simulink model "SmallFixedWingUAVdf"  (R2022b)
settings: Solver=ode4  StartTime=0  StopTime=stoptime  FixedStep=0.001  RelTol=1e-3  EnableMultiTasking=on
PreLoadFcn:
  | asbswarm_vehicledata; % load in workspace variables
PostLoadFcn:
  | open_system([gcs,'/MATLAB Animation Display/MATLAB',10,'Animation']);
InitFcn:
  | InitDatactrl
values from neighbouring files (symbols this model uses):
  uav = struct    [InitDatactrl.m]    (also in InitDatactrldf.m)
undefined symbols (not defined in the file or in its folder): Busy, Wait
libraries: aerolibptmass x1, aerolibanimutils x1

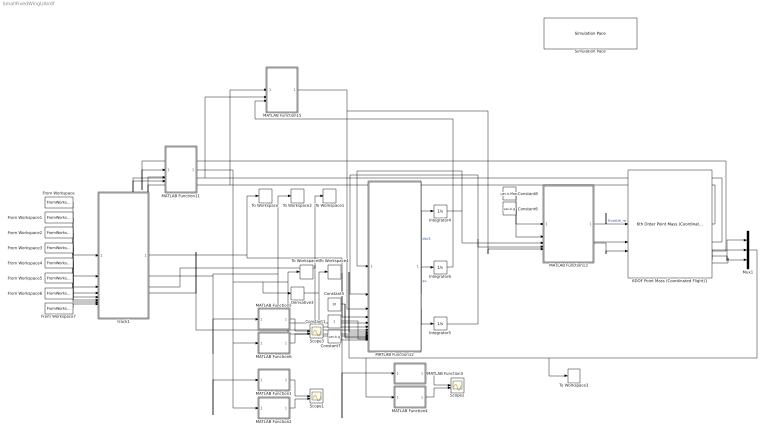
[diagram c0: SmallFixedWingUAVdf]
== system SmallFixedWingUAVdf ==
  6DOF Point Mass (Coordinated Flight)1 : aerolibptmass/6th Order Point Mass (Coordinated Flight)  units=Metric (MKS)  gamma0=uav.ic.Gam  chi0=uav.ic.Chi  V0=uav.ic.V  x0=uav.ic.East  y0=uav.ic.North  h0=uav.ic.Up  mass0=uav.ic.Mass
  Constant1 : Constant
  Constant5 : Constant  Value=10
  Constant6 : Constant  Value=uav.ic.g
  Constant7 : Constant  Value=uav.ic.g
  Constant8 : Constant  Value=uav.ic.Mass
  Derivative3 : Derivative
  From Workspace : FromWorkspace  VariableName=xts  SampleTime=-1
  From Workspace1 : FromWorkspace  VariableName=yts  SampleTime=-1
  From Workspace2 : FromWorkspace  VariableName=dxts  SampleTime=-1
  From Workspace3 : FromWorkspace  VariableName=dyts  SampleTime=-1
  From Workspace4 : FromWorkspace  VariableName=ddxts  SampleTime=-1
  From Workspace5 : FromWorkspace  VariableName=ddyts  SampleTime=-1
  From Workspace6 : FromWorkspace  VariableName=dddxts  SampleTime=-1
  From Workspace7 : FromWorkspace  VariableName=dddyts  SampleTime=-1
  Integrator4 : Integrator
  Integrator5 : Integrator
  Integrator6 : Integrator
  MATLAB Function1 : MATLAB Function  TreatAsAtomicUnit=on
  MATLAB Function11 : MATLAB Function  TreatAsAtomicUnit=on
  MATLAB Function12 : MATLAB Function  TreatAsAtomicUnit=on
  MATLAB Function13 : MATLAB Function  TreatAsAtomicUnit=on
  MATLAB Function15 : MATLAB Function  TreatAsAtomicUnit=on
  MATLAB Function2 : MATLAB Function  TreatAsAtomicUnit=on
  MATLAB Function3 : MATLAB Function  TreatAsAtomicUnit=on
  MATLAB Function4 : MATLAB Function  TreatAsAtomicUnit=on
  MATLAB Function5 : MATLAB Function  TreatAsAtomicUnit=on
  MATLAB Function6 : MATLAB Function  TreatAsAtomicUnit=on
  Mux1 : Mux  Inputs=3
  Scope1 : Scope  NumInputPorts=2
  Scope2 : Scope  NumInputPorts=2
  Scope3 : Scope  NumInputPorts=2
  Simulation Pace : aerolibanimutils/Simulation Pace  SimulationPace=1  SleepMode=Busy-Wait  OutputPaceError=off  SampleTime=-1
  To Workspace : ToWorkspace  VariableName=Xd  SampleTime=0.1
  To Workspace1 : ToWorkspace  VariableName=Ad  SampleTime=0.1
  To Workspace2 : ToWorkspace  VariableName=Vd  SampleTime=0.1
  To Workspace3 : ToWorkspace  VariableName=X  SampleTime=0.1
  To Workspace4 : ToWorkspace  VariableName=A  SampleTime=0.1
  To Workspace5 : ToWorkspace  VariableName=V  SampleTime=0.1
  track1 : MATLAB Function  TreatAsAtomicUnit=on
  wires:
  Constant5/1 -> MATLAB Function12/11(k1), MATLAB Function12/12(k2)
  Constant6/1 -> MATLAB Function13/2(g)
  Integrator5/1 -> MATLAB Function13/4(av3), MATLAB Function12/2(av3)
  MATLAB Function12/1(dav1) -> Integrator4/1  "dav1"
  Integrator4/1 -> MATLAB Function12/1(av1), MATLAB Function13/3(av1)
  Derivative3/1 -> To Workspace4/1, MATLAB Function12/10(ddx)
  MATLAB Function12/3(dav3) -> Integrator5/1
  Constant7/1 -> MATLAB Function12/14(g)
  MATLAB Function13/2(Fy) -> 6DOF Point Mass (Coordinated Flight)1/2
  MATLAB Function13/1(Fx) -> 6DOF Point Mass (Coordinated Flight)1/1  "throttle_re"
  MATLAB Function13/3(Fz) -> 6DOF Point Mass (Coordinated Flight)1/3
  Constant8/1 -> MATLAB Function13/1(m)
  6DOF Point Mass (Coordinated Flight)1/3 -> MATLAB Function11/1(Velocity)
  6DOF Point Mass (Coordinated Flight)1/1 -> MATLAB Function15/1(gamma), MATLAB Function11/2(gamma)
  6DOF Point Mass (Coordinated Flight)1/2 -> MATLAB Function15/2(chi), MATLAB Function11/3(chi)
  MATLAB Function11/1(dx) -> To Workspace5/1, MATLAB Function12/9(dx), Derivative3/1, MATLAB Function6/1(u), MATLAB Function2/1(u)
  MATLAB Function12/2(w1) -> Integrator6/1  "av"
  Integrator6/1 -> MATLAB Function15/3(mu)
  MATLAB Function15/1(R) -> MATLAB Function13/5(R), MATLAB Function12/3(R)
  MATLAB Function5/1(y) -> Scope3/1
  MATLAB Function6/1(y) -> Scope3/2
  MATLAB Function1/1(y) -> Scope1/1
  MATLAB Function2/1(y) -> Scope1/2
  6DOF Point Mass (Coordinated Flight)1/5 -> Mux1/2
  6DOF Point Mass (Coordinated Flight)1/6 -> Mux1/3
  6DOF Point Mass (Coordinated Flight)1/4 -> Mux1/1
  Mux1/1 -> To Workspace3/1, MATLAB Function12/8(x), MATLAB Function4/1(u)
  MATLAB Function4/1(y) -> Scope2/2
  MATLAB Function3/1(y) -> Scope2/1
  From Workspace/1 -> track1/1(x)
  From Workspace1/1 -> track1/2(y)
  From Workspace2/1 -> track1/3(dx)
  From Workspace3/1 -> track1/4(dy)
  From Workspace4/1 -> track1/5(ddx)
  From Workspace5/1 -> track1/6(ddy)
  From Workspace6/1 -> track1/7(dddx)
  From Workspace7/1 -> track1/8(dddy)
  track1/1(Xd) -> To Workspace/1, MATLAB Function12/4(xd), MATLAB Function3/1(u)
  track1/2(Vd) -> To Workspace2/1, MATLAB Function12/5(dxd), MATLAB Function1/1(u), MATLAB Function5/1(u)
  track1/3(Ad) -> To Workspace1/1, MATLAB Function12/6(ddxd)
  track1/4(Jd) -> MATLAB Function12/7(dddxd)
  Constant1/1 -> MATLAB Function12/13(k3)

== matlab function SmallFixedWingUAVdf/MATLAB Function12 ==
function [dav1,w1,dav3] = DF(av1,av3,R,xd,dxd,ddxd,dddxd,x,dx,ddx,k1,k2,k3,g)
    dav1=zeros(1,1);
    w1=zeros(1,1);
    dav3=zeros(1,1);
    
    V = norm(dx,2);
    gv = R'*[0;0;-g];
    w2=-(av3+gv(3))/V;
    w3=gv(2)/V;

    u = dddxd + k1*(ddxd-ddx) + k2*(dxd-dx)+ k3*(xd-x);

    a = [-w2*av3;w3*av1/av3;w2*av1];
    B = [1,0,0;0,-1/av3,0;0,0,1];
    out = a + B*R'*u;

    dav1=out(1); w1=out(2); dav3=out(3);

    if isnan(dav1)
        dav1=0;
    end
    if isnan(w1)
        w1=0;
    end
    if isnan(dav3)
        dav3=0;
    end

end

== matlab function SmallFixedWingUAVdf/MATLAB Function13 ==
function [Fx,Fy,Fz] = fcn(m,g,av1,av3,R)
N=3;
Fxyz=zeros(N,1);

av = [av1;0;av3];
a = [0;0;-g]+R*av;
Fxyz = R'*(m*a);
Fx=Fxyz(1);
Fy=Fxyz(2);
Fz=Fxyz(3);

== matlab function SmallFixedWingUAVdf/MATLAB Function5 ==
function y = fcn(u)

y = u(1);

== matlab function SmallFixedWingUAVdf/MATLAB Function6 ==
function y = fcn(u)

y = u(1);

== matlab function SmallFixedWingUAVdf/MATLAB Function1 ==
function y = fcn(u)

y = u(2);

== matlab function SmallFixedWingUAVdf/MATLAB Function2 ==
function y = fcn(u)

y = u(2);

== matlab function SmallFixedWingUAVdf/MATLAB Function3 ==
function y = fcn(u)

y = u(2);

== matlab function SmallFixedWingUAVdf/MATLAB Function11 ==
function dx = fcn(Velocity,gamma,chi)
 
%     dx(i,:)=[Velocity(i)*cos(gamma(i))*cos(chi(i)),Velocity(i)*sin(gamma(i))*cos(chi(i)),Velocity(i)*sin(gamma(i))];
    dx=[Velocity*cos(chi)*cos(gamma),Velocity*sin(chi)*cos(gamma),Velocity*sin(gamma)]';

end

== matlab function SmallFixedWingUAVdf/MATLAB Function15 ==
function R = fcn(gamma,chi,mu)
    roll = mu;
    pitch = gamma;
    yaw = chi;

    R = ROTZ(yaw)*ROTX(roll)*ROTY(pitch);
end

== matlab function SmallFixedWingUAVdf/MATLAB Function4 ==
function y = fcn(u)

y = u(2);

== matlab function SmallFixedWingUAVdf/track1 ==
function [Xd,Vd,Ad,Jd] = fcn(x,y,dx,dy,ddx,ddy,dddx,dddy)
    Xd = [x,y,100]';
    Vd = [dx,dy,0]';
    Ad = [ddx,ddy,0]';
    Jd = [dddx,dddy,0]';
end
